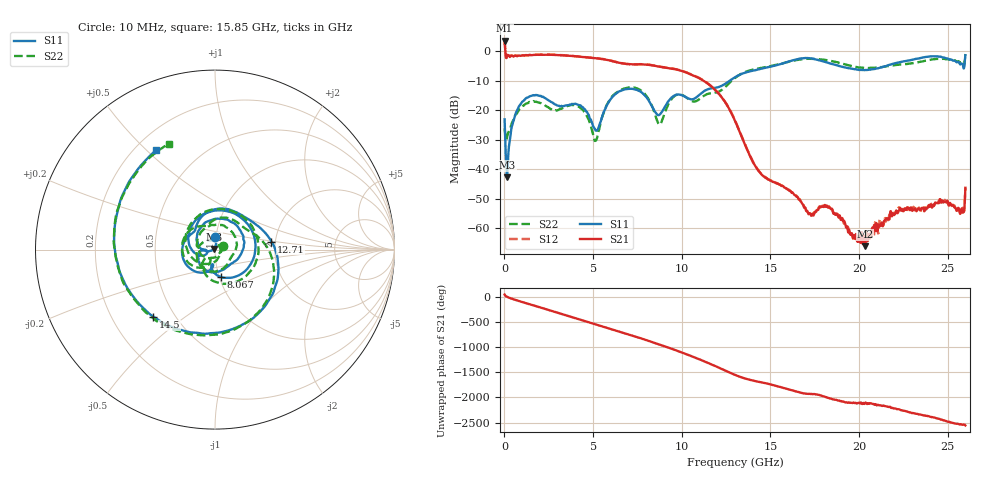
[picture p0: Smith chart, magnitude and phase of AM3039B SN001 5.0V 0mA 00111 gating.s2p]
!Agilent Technologies,E8364B,MY43040894,A.07.50.67
!Agilent E8364B: A.07.50.67
!Date: Tuesday, June 28, 2016 08:04:49
!Correction: S11(Full 2 Port(1,2))
!S21(Full 2 Port(1,2))
!S12(Full 2 Port(1,2))
!S22(Full 2 Port(1,2))
!S2P File: Measurements: S11, S21, S12, S22:
# Hz S  dB  R 50
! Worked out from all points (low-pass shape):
!   1601 points, 10 MHz to 26 GHz, reference 50 ohm
!   highest |S21| = 3.62 dB at 10 MHz (marker M1); lowest = -66.2 dB at 20.33 GHz (marker M2)
!   |S21| within 3 dB of the highest: start of sweep to 44.36 MHz
!   lowest |S11| = -42.8 dB at 156.2 MHz (marker M3), VSWR 1.01, Z = 49.4 + j0.335 ohm
!   |S11| at or under -10 dB: start of sweep to 12.7 GHz
!   |S22| runs from -30.4 to -0.9 dB; largest |S21 - S12| = 0.026
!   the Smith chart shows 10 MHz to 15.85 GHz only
!   S11 on the Smith chart (normalised r, x): 10 MHz: 0.99, +0.14; 8.067 GHz: 1.02, -0.32; 12.71 GHz: 1.91, +0.19; 14.5 GHz: 0.38, -0.38; 15.85 GHz: 0.28, +0.54
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1e7  -23.09 88.4  3.62 40.6  3.69 41.5  -26.19 20.7
1.561938e8  -42.84 151.9  -1.40 -5.4  -1.33 -5.2  -28.93 -63.7
1.618131e9  -14.90 69.2  -1.22 -172.7  -1.17 -172.6  -16.96 74.9
2.495294e9  -16.67 -10.1  -1.17 95.1  -1.11 95.2  -19.12 -7.6
3.291238e9  -18.64 -54.8  -1.36 10.7  -1.30 10.9  -19.24 -54.7
4.347081e9  -18.75 -138.3  -1.89 -102.5  -1.86 -102.4  -19.54 -165.5
5.792775e9  -18.14 -176.1  -2.92 98.8  -2.87 99.1  -17.93 -151.3
6.7674e9  -12.98 72.0  -4.22 -6.1  -4.16 -5.9  -12.61 69.1
8.0669e9  -16.07 -77.2  -4.54 -150.5  -4.48 -150.1  -15.66 -100.0
8.684162e9  -21.69 -99.8  -5.14 136.2  -5.07 136.6  -24.53 -131.3
1.271261e10  -9.95 8.1  -19.96 -67.6  -19.79 -67.1  -10.60 1.1
1.3005e10  -8.80 -13.7  -23.59 -112.3  -23.46 -112.0  -9.05 -20.8
1.449942e10  -5.89 -132.5  -41.80 98.6  -41.68 98.6  -5.63 -142.9
1.584766e10  -3.82 120.4  -46.38 -21.6  -46.28 -22.3  -3.84 113.8
1.734208e10  -2.46 -19.3  -55.37 -130.5  -55.64 -129.7  -2.53 -12.4
1.886899e10  -4.97 -152.1  -56.01 99.9  -56.56 96.6  -3.92 -141.2
2.033093e10  -6.34 103.8  -66.16 44.0  -64.43 40.5  -5.64 113.1
2.167916e10  -4.65 13.6  -56.85 -30.1  -56.07 -22.9  -5.00 19.4
2.309237e10  -2.75 -92.4  -53.68 -153.2  -52.94 -154.6  -3.96 -82.7
2.419694e10  -1.65 178.1  -52.34 122.5  -52.02 124.0  -2.69 -167.0
2.515532e10  -2.75 95.8  -51.66 26.1  -51.86 25.4  -2.83 112.5
2.6e10  -1.35 -24.2  -46.33 -35.3  -46.27 -40.1  -0.91 4.3
